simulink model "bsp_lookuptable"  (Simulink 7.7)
settings: Solver=ode45  StartTime=0.0  StopTime=20.0  RelTol=1e-3
PreLoadFcn:
  | bsp_lookuptable_ini
InitFcn:
  | bsp_lookuptable_ini
StopFcn:
  | bsp_lookuptable_plot
libraries: simulink x1

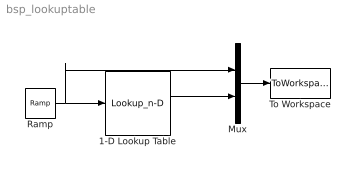
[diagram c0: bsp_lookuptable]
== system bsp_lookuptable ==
  1-D Lookup Table : Lookup_n-D  NumberOfTableDimensions=1  BreakpointsForDimension1=[-10,-8,-6,-4,-2,0,2,4,6,8,10]  Table=[-5,-5,-5,-2,-2,-2,4.5,4.5,4.5,0,-1]  RndMeth=Simplest
  Mux : Mux  Inputs=2
  Ramp : simulink/Sources/Ramp  SystemSampleTime=-1  slope=1  start=0  X0=-10
  To Workspace : ToWorkspace  VariableName=auslese  SampleTime=-1  SaveFormat=Array
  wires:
  1-D Lookup Table/1 -> Mux/2
  Ramp/1 -> Mux/1, 1-D Lookup Table/1
  Mux/1 -> To Workspace/1
